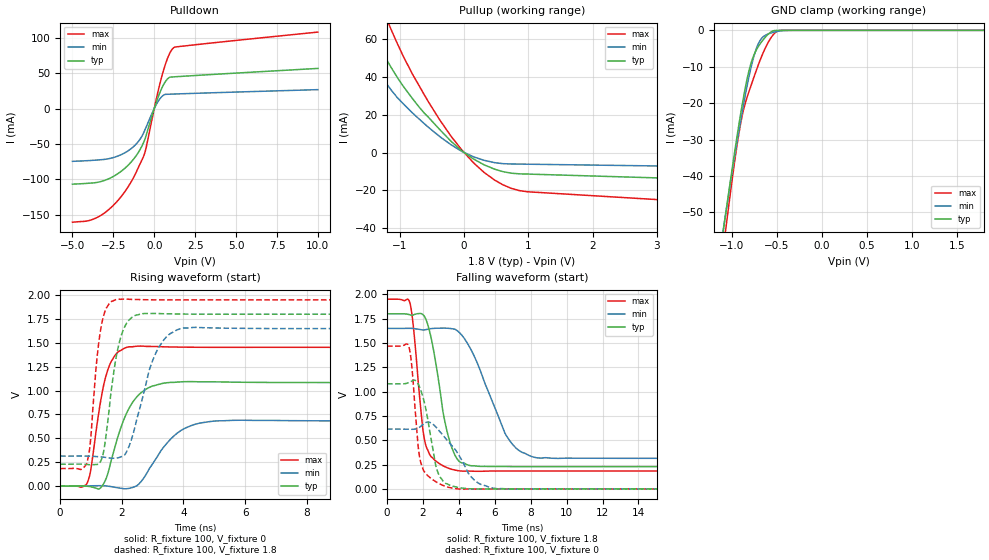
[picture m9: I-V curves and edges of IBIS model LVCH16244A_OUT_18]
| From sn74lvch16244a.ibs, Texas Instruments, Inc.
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[Model]   LVCH16244A_OUT_18
Model_type  3-state
Enable   Active-Low
Vref =   0
Rref =   1000
Cref =   30p
Vmeas =   0.9
| variable   typ   min   max
C_comp   5.05pF   4.64pF   6.06pF
| C_pullup   8.51pF   3.38pF   19.85pF
| C_pulldown   8.29pF   5.63pF   10.77pF
| C_tri-state   5.05pF   4.64pF   6.06pF
[Temperature Range]   40   100   -40
| Ambient temperature   25   85   -40
[Voltage range]   1.8   1.65   1.95
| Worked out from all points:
|   slope of the pulldown table from 0 to 0.27 V, typ, clamps not added: 14.8 ohm
|   slope of the pullup table from 0 to 0.27 V, typ, clamps not added: 46.7 ohm
|   GND clamp passes 1 mA (typ) near -0.59 V on its own axis
|   rising waveform, R_fixture 100, V_fixture 0: 20-80 % time 714ps typ, 948ps min, 446ps max; typ from 0 V to 1.08 V
|   falling waveform, R_fixture 100, V_fixture 1.8: 20-80 % time 880ps typ, 1.74ns min, 551ps max; typ from 1.8 V to 0.23 V
|   rising waveform, R_fixture 100, V_fixture 1.8: 20-80 % time 413ps typ, 693ps min, 292ps max; typ from 0.229 V to 1.8 V
|   falling waveform, R_fixture 100, V_fixture 0: 20-80 % time 642ps typ, 1.3ns min, 428ps max; typ from 1.08 V to 0 V
[GND Clamp]
| LVCH16244A_OUT_18
|   Voltage   I(typ)   I(min)   I(max)
-5V       -855.7mA   -797.6mA   -953.2mA
-1.085V   -53.47mA   -53.15mA   -58.22mA
-1.06V    -49.06mA   -49.09mA   -53.29mA
-975mV    -34.56mA   -35.69mA   -37.29mA
-910mV    -24.24mA   -26.03mA   -26.76mA
-865mV    -17.79mA   -19.78mA   -21.4mA
-800mV    -10.27mA   -11.72mA   -16.17mA
-740mV    -6.037mA   -5.97mA    -11.9mA
-685mV    -3.711mA   -2.772mA   -8.196mA
-590mV    -945.4uA   -940.9uA   -3.072mA
-510mV    -31.84uA   -379.7uA   -498.3uA
1.8V      7.563pA    17.53nA    3.673pA
[Pulldown]
| LVCH16244A_OUT_18
|   Voltage   I(typ)   I(min)   I(max)
-5V       -106.8mA   -74.48mA   -160.5mA
-3.945V   -105.3mA   -73.35mA   -157.9mA
-3.11V    -102mA     -71.9mA    -148.6mA
-2.21V    -91.71mA   -66.9mA    -129.5mA
-1.4V     -75.15mA   -56.3mA    -103.1mA
-920mV    -59.95mA   -44.93mA   -80.72mA
-585mV    -44.32mA   -30.88mA   -63.04mA
60mV      4.341mA    2.845mA    6.529mA
455mV     28.54mA    16.86mA    44.89mA
845mV     42.74mA    20.36mA    72.96mA
1.185V    44.91mA    20.64mA    86.07mA
10V       56.83mA    26.86mA    108.2mA
[Pullup]
| LVCH16244A_OUT_18
|   Voltage   I(typ)   I(min)   I(max)
-5V       29.31mA    10.34mA    78.9mA
-3.56V    38.96mA    11.4mA     214.8mA
-3.24V    48.87mA    12.22mA    244.5mA
-3.11V    69.83mA    12.77mA    236.3mA
-2.795V   142.2mA    15.56mA    212.5mA
-2.62V    134.9mA    22.74mA    198mA
-2.515V   129.6mA    70.32mA    189mA
-1.885V   92.49mA    69.08mA    132.8mA
-1.13V    44.7mA     32.87mA    64.59mA
-35mV     915.1uA    617uA      1.397mA
860mV     -11.22mA   -6.065mA   -20.08mA
10V       -20.36mA   -10.29mA   -39.14mA
[Ramp]
| LVCH16244A_OUT_18
| variable   typ   min   max
dV/dt_r   0.67/7.50E-10   0.43/1.05E-09   0.88/4.61E-10
dV/dt_f   0.94/9.56E-10   0.80/1.80E-09   1.06/5.88E-10
R_load = 100
[Rising Waveform]
| LVCH16244A_OUT_18
R_fixture =   100
C_fixture =   0
L_fixture =   0
V_fixture =   0
V_fixture_min = 0
V_fixture_max = 0
|   Time   V(typ)   V(min)   V(max)
0s        -30.55uV   -44.63uV   -15.38uV
865ps     -790.5uV   1.982mV    23.06mV
1.25ns    -31.85mV   4.405mV    762.8mV
1.51ns    95.17mV    1.511mV    1.18V
1.82ns    458.1mV    -14.81mV   1.385V
2.25ns    823.4mV    -22.57mV   1.459V
2.86ns    1.028V     162.8mV    1.463V
3.81ns    1.089V     557.6mV    1.456V
5.115ns   1.091V     683.4mV    1.453V
49.99ns   1.085V     680.7mV    1.454V
[Falling Waveform]
| LVCH16244A_OUT_18
R_fixture =   100
C_fixture =   0
L_fixture =   0
V_fixture =   1.8
V_fixture_min = 1.65
V_fixture_max = 1.95
|   Time   V(typ)   V(min)   V(max)
0s        1.8V       1.65V      1.95V
1.28ns    1.79V      1.651V     1.91V
2.13ns    1.758V     1.636V     471.4mV
2.55ns    1.469V     1.649V     317.3mV
3.28ns    644.2mV    1.653V     223.8mV
3.865ns   320.1mV    1.632V     190.8mV
4.835ns   237.8mV    1.374V     181.9mV
6.685ns   229.9mV    536.4mV    183.9mV
8.335ns   229.2mV    320mV      184.1mV
49.99ns   229.5mV    314.9mV    184mV
[Rising Waveform]
| LVCH16244A_OUT_18
R_fixture =   100
C_fixture =   0
L_fixture =   0
V_fixture =   1.8
V_fixture_min = 1.65
V_fixture_max = 1.95
|   Time   V(typ)   V(min)   V(max)
0s        229.5mV    314.8mV    184mV
865ps     226.6mV    314.4mV    238.1mV
970ps     224mV      313.6mV    426.3mV
1.31ns    257.6mV    306.1mV    1.631V
1.505ns   573mV      299mV      1.867V
1.87ns    1.436V     295.8mV    1.957V
2.26ns    1.746V     438.2mV    1.955V
3.14ns    1.808V     1.417V     1.95V
4.025ns   1.801V     1.656V     1.95V
49.99ns   1.8V       1.65V      1.95V
[Falling Waveform]
| LVCH16244A_OUT_18
R_fixture =   100
C_fixture =   0
L_fixture =   0
V_fixture =   0
V_fixture_min = 0
V_fixture_max = 0
|   Time   V(typ)   V(min)   V(max)
0s        1.081V     614.9mV    1.468V
1.215ns   1.093V     613.5mV    1.462V
1.39ns    1.109V     612.9mV    1.247V
1.69ns    1.094V     622.1mV    539mV
2.03ns    926.1mV    666.5mV    193.8mV
2.83ns    172.3mV    614.7mV    61.97mV
3.765ns   24.01mV    413.2mV    4.616mV
4.84ns    21.56uV    95.11mV    -1.335mV
6.145ns   75.89uV    2.771mV    36.5uV
49.99ns   314.7nV    22.2uV     -801.1nV
